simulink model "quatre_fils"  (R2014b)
settings: Solver=ode45  StartTime=0.0  StopTime=10.0  RelTol=1e-3
libraries: elec_lib x6, fl_lib x2, nesl_utility x2

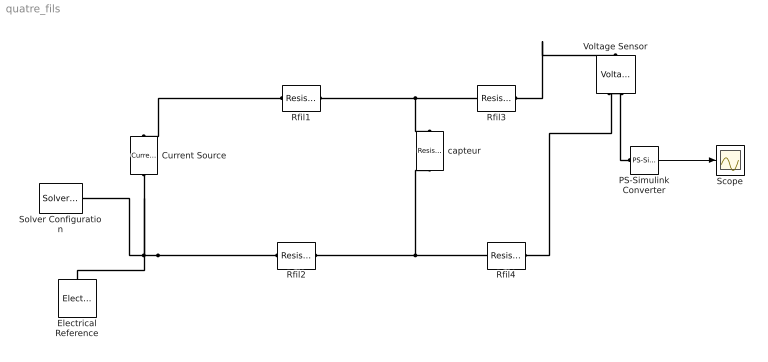
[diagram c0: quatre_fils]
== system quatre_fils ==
  Current Source : elec_lib/Sources/Current Source  dc_current=0.01 A  ac_current=0 A  ac_shift=0 deg  ac_frequency=60 Hz  noise_mode=0  PSD=0 A^2/Hz  sample_time=0.001 s  repeatability=1  auto_seed=3922919431  user_seed=0
  Electrical Reference : fl_lib/Electrical/Electrical Elements/Electrical Reference
  PS-Simulink Converter : nesl_utility/PS-Simulink Converter  PhysicalDomain=network_engine_domain  SubClassName=ps_output  LeftPortType=input  RightPortType=output  PseudoPeriodic=off  Frequencies=[]  Unit=1  AffineConversion=off
  Rfil1 : elec_lib/Passive Devices/Resistor  R=1.5 Ohm  noise_mode=0  Tdevice=25 C  sample_time=0.001 s  repeatability=1  auto_seed=3890346746  user_seed=0
  Rfil2 : elec_lib/Passive Devices/Resistor  R=3 Ohm  noise_mode=0  Tdevice=25 C  sample_time=0.001 s  repeatability=1  auto_seed=3499211588  user_seed=0
  Rfil3 : elec_lib/Passive Devices/Resistor  R=1 Ohm  noise_mode=0  Tdevice=25 C  sample_time=0.001 s  repeatability=1  auto_seed=1030588251  user_seed=0
  Rfil4 : elec_lib/Passive Devices/Resistor  R=1 Ohm  noise_mode=0  Tdevice=25 C  sample_time=0.001 s  repeatability=1  auto_seed=1792148415  user_seed=0
  Scope : Scope
  Solver Configuration : nesl_utility/Solver Configuration  PhysicalDomain=network_engine_domain  SubClassName=solver  LeftPortType=input  RightPortType=generic  Accelerate=off  Tones=[]  Harmonics=[]  SimulateNoise=off  Profile=off  UseLocalSampling=off  EnableSwitchedLinearOptims=on  FrequencyDomain=off  UseCCode=off  RelTol=0.001  AbsTol=1e-06  MinStep=1e-09  ToWorkspace=off  DoDC=off  ResidualTolerance=1e-09  UseLocalSolver=off  LocalSolverChoice=NE_BACKWARD_EULER_ADVANCER  LocalSolverSampleTime=0.001  DoFixedCost=off  MaxNonlinIter=3  MaxModeIter=2  LinearAlgebra=Sparse  DelaysMemoryBudget=1024  AutomaticFiltering=on  FilteringTimeConstant=0.001
  Voltage Sensor : fl_lib/Electrical/Electrical Sensors/Voltage Sensor
  capteur : elec_lib/Passive Devices/Resistor  R=100 Ohm  noise_mode=0  Tdevice=25 C  sample_time=0.001 s  repeatability=1  auto_seed=545404223  user_seed=0
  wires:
  PS-Simulink Converter/1 -> Scope/1
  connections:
  Rfil1/RConn1 -- Rfil3/LConn1 -- capteur/LConn1
  Rfil2/LConn1 -- Electrical Reference/LConn1 -- Solver Configuration/RConn1 -- Current Source/RConn1
  Rfil1/LConn1 -- Current Source/LConn1
  PS-Simulink Converter/LConn1 -- Voltage Sensor/RConn1
  Rfil2/RConn1 -- Rfil4/LConn1 -- capteur/RConn1
  Rfil3/RConn1 -- Voltage Sensor/LConn1
  Rfil4/RConn1 -- Voltage Sensor/RConn2
